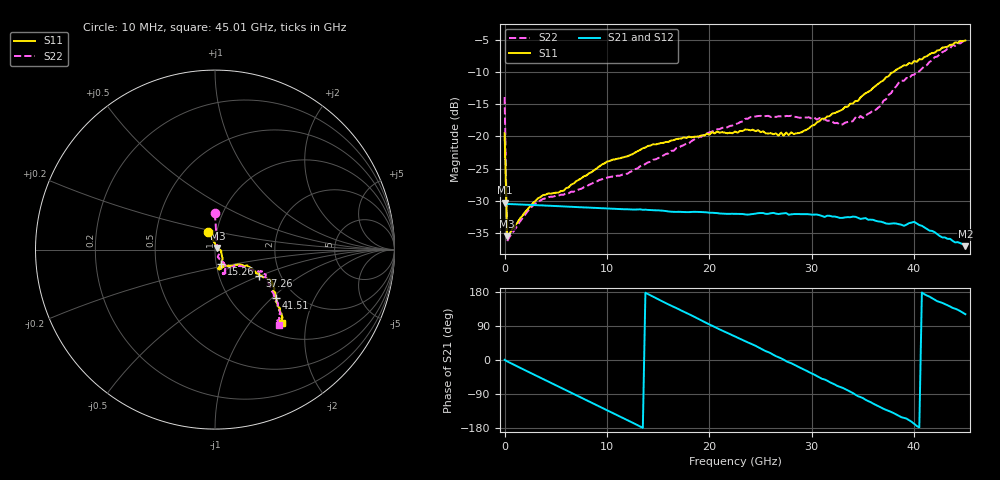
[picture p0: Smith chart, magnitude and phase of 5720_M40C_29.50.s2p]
! Device:  ADRF5720
! Description: 0.5dB LSB GaAs MMIC 6-bit Digital Attenuator
! Frequency:  0.000009 -  40 GHz
! Ports:
!	RF1	= Port 1
!	RF2	= Port 2
! Vdd:  3.3 Volt
! Vss:  -3.3 Volt
! Control:  0/3.3 Volt
! State:  29.50 dB attenuation
! Data:  The device was measured using G-S-G Probes on a matrix board.
!  Data was collected using an calibrated 4 port network analyzer.
!  The reference plane for this measurement is at the launchers.
! Note:  Analog Devices supplies this data as a sample of measured data
!  for this product.  Your particular data for this product may vary.
!  Data was taken at -40 degrees C.
!  Analog Devices reserves the right to change this data at anytime.
# GHZ S DB R 45.0
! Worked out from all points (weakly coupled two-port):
!   181 points, 10 MHz to 45.01 GHz, reference 45 ohm
!   highest |S21| = -30.29 dB at 10 MHz (marker M1); lowest = -37.0 dB at 45.01 GHz (marker M2)
!   lowest |S11| = -35.5 dB at 260 MHz (marker M3), VSWR 1.03, Z = 46.3 + j0.884 ohm
!   |S11| at or under -10 dB: start of sweep to 38.01 GHz
!   |S22| runs from -36.2 to -5.2 dB; largest |S21 - S12| = 0.00014
!   S11 on the Smith chart (normalised r, x): 10 MHz: 0.91, +0.18; 15.26 GHz: 1.06, -0.17; 37.26 GHz: 1.56, -0.50; 41.51 GHz: 1.60, -1.06; 45.01 GHz: 1.24, -1.46
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0.01  -19.53 112.3  -30.29 0.5  -30.33 0.5  -13.89 90.3
0.26  -35.50 34.7  -30.48 -3.6  -30.50 -3.7  -36.24 32.4
3.26  -29.60 -8.9  -30.67 -43.6  -30.70 -43.6  -30.07 -32.6
5.76  -28.43 -25.0  -30.85 -76.4  -30.87 -76.4  -29.04 -52.5
7.76  -26.18 -39.2  -31.01 -102.7  -31.02 -102.7  -27.88 -65.7
10.01  -23.91 -48.2  -31.18 -132.4  -31.19 -132.5  -26.40 -67.6
12.01  -23.09 -56.0  -31.30 -158.9  -31.32 -159.0  -25.78 -66.1
15.26  -21.03 -66.5  -31.49 156.8  -31.51 156.8  -23.20 -59.6
20.26  -19.33 -77.8  -31.84 90.7  -31.86 90.6  -19.25 -57.9
22.76  -19.41 -80.2  -32.03 58.9  -32.05 58.8  -18.00 -63.6
24.01  -19.06 -75.2  -32.08 43.7  -32.11 43.6  -17.00 -64.8
27.26  -19.89 -65.7  -31.93 0.9  -31.96 0.8  -16.96 -69.0
30.26  -18.23 -47.0  -32.12 -38.7  -32.13 -38.8  -17.09 -70.5
33.01  -15.84 -31.0  -32.63 -73.4  -32.66 -73.5  -18.14 -55.6
35.01  -13.61 -27.4  -32.72 -100.6  -32.74 -100.8  -17.15 -40.4
37.26  -10.82 -30.5  -33.50 -131.5  -33.51 -131.6  -14.23 -31.6
37.76  -10.16 -30.0  -33.52 -137.1  -33.56 -137.1  -13.28 -30.3
38.76  -9.22 -28.4  -33.69 -150.9  -33.72 -151.1  -11.33 -27.0
40.01  -8.29 -31.6  -33.25 -168.4  -33.29 -168.5  -10.41 -26.4
41.51  -7.27 -38.2  -34.61 167.1  -34.64 166.9  -8.44 -34.8
43.76  -5.78 -43.9  -36.19 137.6  -36.22 137.1  -5.79 -44.4
45.01  -5.12 -47.5  -37.02 120.8  -37.02 120.8  -5.23 -49.7
